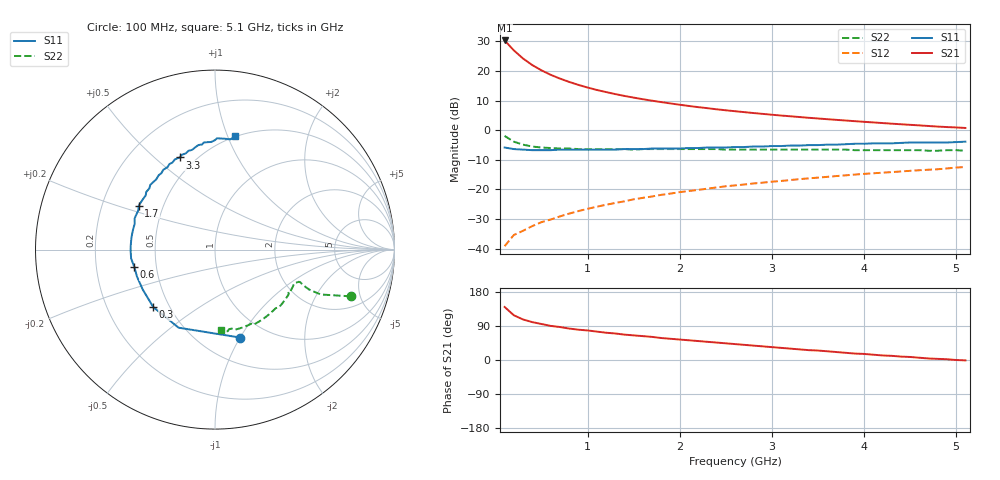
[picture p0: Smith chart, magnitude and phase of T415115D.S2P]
!AT-41511
!S-PARAMETERS at Vce=5V  Ic=25mA.  LAST UPDATED 01-25-95
# ghz s ma r 50
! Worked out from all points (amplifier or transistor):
!   51 points, 100 MHz to 5.1 GHz, reference 50 ohm
!   highest |S21| = 30.3 dB at 100 MHz (marker M1)
!   |S21| within 3 dB of that: start of sweep to 189.7 MHz
!   unconditionally stable (mu >= 1): 574.1 MHz to 3.189 GHz
!   at 900 MHz: K = 1.10, MAG = 19.4 dB, |S12| = -27.3 dB
!   at 2.6 GHz: K = 1.06, MAG = 11.0 dB, |S12| = -18.6 dB
!   at 5.1 GHz: K = 0.85, MSG = 6.6 dB, |S12| = -12.4 dB
!   lowest NFmin = 1.60 dB at 100 MHz
!   S11 on the Smith chart (normalised r, x): 100 MHz: 0.76, -1.00; 300 MHz: 0.41, -0.34; 600 MHz: 0.37, -0.09; 1.7 GHz: 0.36, +0.23; 3.3 GHz: 0.41, +0.61; 5.1 GHz: 0.50, +1.06
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0.1  0.51 -74.0  32.79 140.0  0.011 65.0  0.8 -19.0
0.2  0.48 -115.0  22.31 118.0  0.017 57.0  0.64 -23.0
0.3  0.47 -137.0  16.24 107.0  0.02 58.0  0.57 -23.0
0.4  0.46 -151.0  12.59 100.0  0.024 59.0  0.53 -22.0
0.5  0.46 -161.0  10.26 95.0  0.028 62.0  0.51 -21.0
0.6  0.46 -168.0  8.616 90.0  0.031 63.0  0.5 -21.0
0.7  0.47 -174.0  7.445 87.0  0.035 65.0  0.49 -22.0
0.8  0.47 -179.0  6.544 83.0  0.039 66.0  0.49 -22.0
0.9  0.47 177.0  5.83 80.0  0.043 66.0  0.48 -23.0
1  0.47 173.0  5.257 78.0  0.047 67.0  0.48 -24.0
1.1  0.47 170.0  4.787 75.0  0.051 68.0  0.48 -25.0
1.2  0.47 166.0  4.413 72.0  0.055 68.0  0.48 -26.0
1.3  0.47 162.0  4.076 70.0  0.059 68.0  0.48 -28.0
1.5  0.48 157.0  3.553 65.0  0.068 68.0  0.47 -30.0
1.7  0.49 150.0  3.15 61.0  0.076 68.0  0.48 -32.0
1.8  0.49 148.0  2.983 58.0  0.081 68.0  0.48 -34.0
2.2  0.5 137.0  2.452 50.0  0.098 66.0  0.48 -39.0
2.6  0.52 127.0  2.093 42.0  0.117 64.0  0.47 -45.0
3.3  0.55 111.0  1.669 28.0  0.149 59.0  0.47 -55.0
3.5  0.56 107.0  1.577 25.0  0.158 58.0  0.47 -58.0
4.3  0.6 92.0  1.289 11.0  0.196 52.0  0.46 -71.0
5.1  0.64 80.0  1.091 -1.0  0.239 46.0  0.45 -86.0
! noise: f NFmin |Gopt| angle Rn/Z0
0.1  1.6  0.08  14  0.18
0.9  1.9  0.11  165  0.16
1.8  2.3  0.28  -153  0.18
2.4  2.7  0.39  -134  0.22
